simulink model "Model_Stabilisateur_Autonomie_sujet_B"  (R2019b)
settings: Solver=ode23tb  StartTime=0.0  StopTime=7200  MaxStep=0.1  RelTol=1e-4  EnableMultiTasking=on
undefined symbols (not defined in the file): Ion, Lithium
libraries: powerlib x2, electricdrivelib x1, simulink x1

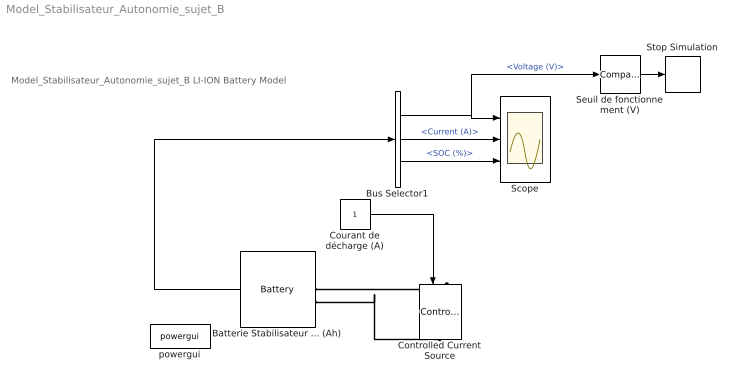
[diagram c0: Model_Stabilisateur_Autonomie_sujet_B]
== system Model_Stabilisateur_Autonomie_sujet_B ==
  note: Model_Stabilisateur_Autonomie_sujet_B LI-ION Battery Model
  Batterie Stabilisateur ... (Ah) : electricdrivelib/Extra Sources/Battery  BatType=Lithium-Ion  ShowTempParam=off  ThermalPreset=no  ShowAgeParam=off  NomV=7.2  NomQ=5.4  SOC=100  Batt_Tr=30  PresetModel=on  MaxQ=5.4  MinV=5.4  FullV=8.3807  Dis_rate=2.3478  R=0.013333  Normal_OP=4.8835  expZone="[7.7788      0.2653]"  current=[6.5 13 32.5]  Units=Time  Tci=20  NomT=20  T2=-30  MaxQ2=4.8  FullV2=7.1  Normal_OP2=5.655  expZone2="[6.58           1]"  Rca=0.6  ti=2000  Dp=0  Neq0=0  Tsim=1e6  Ta1=25  Qeol=5.4*0.9  Reol=0.013333*1.2  Char_age=[2.3478, 3]  Dis_age=[2.3478, 10]  N1=1500  N2=10500  N3=1000  N4=1400  Ta2=45  N5=950
  Bus Selector1 : BusSelector  OutputSignals=Voltage (V),Current (A),SOC (%)
  Controlled Current Source : powerlib/Electrical Sources/Controlled Current Source  Initialize=on  Source_Type=AC  Amplitude=0  Phase=0  Frequency=0  Measurements=None
  Courant de décharge (A) : Constant
  Scope : Scope  NumInputPorts=3
  Seuil de fonctionnement (V) : simulink/Logic and Bit Operations/Compare To Constant  relop=<=  const=1  OutDataTypeStr=boolean
  Stop Simulation : Stop
  powergui : powerlib/powergui  SimulationMode=Continuous  SampleTime=0.001  frequency=60  Iterations=50  frequencyindice=0  Pbase=100e6  ErrMax=1e-4  UnitsV=kV  UnitsW=MW  buscounter=0  FunctionMessages=off  echomessages=off  EnableUseOfTLC=off  CurrentSourceSwitches=off  DisableSnubberDevices=off  DisableRonSwitches=off  DisableVfSwitches=off  DisplayEquations=off  AutomaticDiscreteSolvers=off  SolverType=Tustin  Interpol=off  ExternalGateDelay=off  methode=off  Ts=0  x0status=blocks  SPID=off  SwTol=0  HookPort=off  NonlinearTolerance=1e-4  nMaxIteration=100  ContinueOnMaxIteration=off  RestoreLinks=warning  ResistiveCurrentMeasurement=off  Frange=[0:2:500]  Ylog=off  Xlog=on  ShowGrid=off  save=off  variable=ZData  structure=0  ZoomFFT=on  StartTime=0.0  cycles=1  DisplayStyle=1  fundamental=60  FreqAxis=off  MaxFrequency=1000  frequencyindicesteady=1  RmsSteady=1  display=off
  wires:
  Courant de décharge (A)/1 -> Controlled Current Source/1
  Batterie Stabilisateur ... (Ah)/1 -> Bus Selector1/1
  Bus Selector1/3 -> Scope/3  "<SOC (%)>"
  Bus Selector1/2 -> Scope/2  "<Current (A)>"
  Bus Selector1/1 -> Seuil de fonctionnement (V)/1, Scope/1  "<Voltage (V)>"
  Seuil de fonctionnement (V)/1 -> Stop Simulation/1
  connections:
  Controlled Current Source/RConn1 -- Batterie Stabilisateur ... (Ah)/LConn2
  Controlled Current Source/LConn1 -- Batterie Stabilisateur ... (Ah)/LConn1
